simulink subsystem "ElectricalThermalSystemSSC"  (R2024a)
settings: Solver=VariableStepAuto  StartTime=0.0  StopTime=10.0  RelTol=1e-3
undefined symbols (not defined in the file): coolant_pipe_D, coolant_valve_D_ratio_max, coolant_valve_D_ratio_min, coolant_valve_displacement, EnvAirTemp, EnvGrvty, PlantThrEstCmpPwr, PlntThrChArea, PlntThrFanMaxSpd, PlntThrFanMechEff, PlntThrFanVolEff, PlntThrHeaterMaxPwr, PlntThrPipeArea, PlntThrPipeDia, PlntThrPmpMaxSpd, PlntThrRadRamEff, PlntThrRefrigAinit, PlntThrTankArea, PlntThrTankVol, PlntThrValDisp, PlntThrValDratioMax, PlntThrValDratioMin, PlntThrValSplMax, ThrmEM1, ThrmEM2, ThrmEM3, ThrmEM4
libraries: fl_lib x148, nesl_utility x61, SimscapeFluids_lib x25, autolibutils x12
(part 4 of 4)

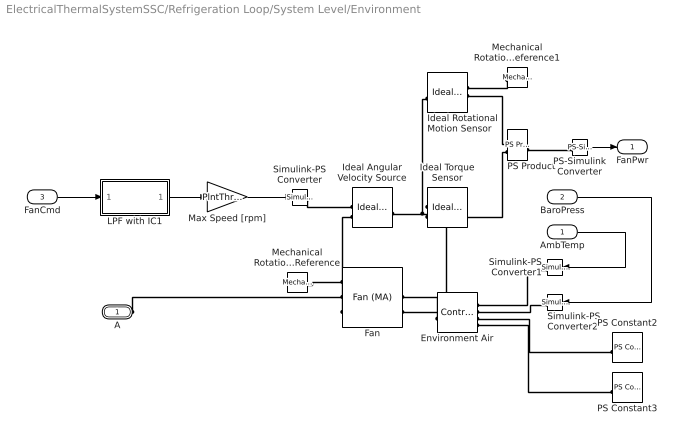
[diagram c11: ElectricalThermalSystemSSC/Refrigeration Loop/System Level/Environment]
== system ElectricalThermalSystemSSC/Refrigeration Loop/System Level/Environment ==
  AmbTemp : Inport
  BaroPress : Inport  Port=2
  FanCmd : Inport  Port=3
  Environment Air : fl_lib/Moist Air/Elements/Controlled Reservoir (MA)  moisture_spec=foundation.enum.moisture_spec.relative_humidity  trace_gas_spec=foundation.enum.trace_gas_spec.mole_fraction  RH_ws=1  area_A=PlntThrRadFanAreaFlw m^2  input_error_spec=foundation.enum.input_range_error.warn
  Fan : SimscapeFluids_lib/Moist Air/Turbomachinery/Fan (MA)  fan_parameterization=fluids.moist_air.turbomachinery.enum.FanParameterization.Nominal  mechanical_power_spec=fluids.moist_air.turbomachinery.enum.FanMechanicalPowerSpec.Efficiency  flow_rate_nominal=0.8 m^3/s  pressure_nominal=PlntThrFanNomP Pa  eta_nominal=PlntThrFanVolEff*PlntThrFanMechEff  power_nominal=1620 W  pressure_max=600 Pa  flow_rate_max=1.5 m^3/s  omega_ref_nominal=1000 rpm  flow_rate_1D_TLU=[.0278, .0556, .0833, .111, .139, .167] m^3/s  pressure_1D_TLU=[6410, 6375, 6018, 5366, 4501, 3609] Pa  eta_1D_TLU=[.257, .394, .453, .47, .459, .415]  power_1D_TLU=[693, 900, 1107, 1267, 1363, 1452] W  omega_ref_1D=3000 rpm  rho_ref_1D=1.2 kg/m^3  omega_threshold_factor=1e-2  omega_dp_TLU=[2400; 3000; 3600] rpm  flow_rate_dp_TLU=[.0278, .0556, .0833, .111, .139, .167] m^3/s  pressure_dp_TLU=[4111, 4010, 3551, 2881, 2167, 1453; 6410, 6375, 6018, 5366, 4501, 3609; 9217, 9285, 9022, 8428, 7552, 6482] Pa  eta_dp_TLU=[.3, .434, .468, .459, .4, .3; .257, .394, .453, .47, .459, .415; .225, .359, .434, .461, .47, .459]  power_dp_TLU=[381, 514, 632, 697, 753, 809; 693, 900, 1107, 1267, 1363, 1452; 1139, 1438, 1732, 2029, 2233, 2358] W  rho_ref_dp=1.2 kg/m^3  omega_q_TLU=[2990; 3450; 3867] rpm  pressure_q_TLU=[31, 62, 93, 124] Pa  flow_rate_q_TLU=[.802, .759, .703, .611; .936, .902, .862, .81; 1.056, 1.027, .994, .956] m^3/s  eta_q_TLU=[.088, .162, .22, .261; .068, .128, .18, .222; .055, .105, .148, .188]  power_q_TLU=[283, 290, 297, 290; 427, 437, 445, 452; 595, 606, 625, 631] W  rho_ref_q=1.2 kg/m^3  diameter_ratio=1  mech_orientation=fluids.moist_air.turbomachinery.enum.FanMechanicalOrientation.Positive  area_A=PlntThrRadFanAreaFlw m^2  area_B=PlntThrRadFanAreaFlw m^2
  Ideal Angular Velocity Source : fl_lib/Mechanical/Mechanical Sources/Ideal Angular Velocity Source
  Ideal Rotational Motion Sensor : fl_lib/Mechanical/Mechanical Sensors/Ideal Rotational Motion Sensor  reference=foundation.enum.MeasurementReference.difference  acceleration_port=false  velocity_port=true  position_port=true  wrap_angle=false  offset=0 rad
  Ideal Torque Sensor : fl_lib/Mechanical/Mechanical Sensors/Ideal Torque Sensor
  LPF with IC1 : Subsystem  mask{wc=0.2, InitCond=0, dataType=off}
      mask prompts: wc "Cutoff frequency, wc [rad/s]"; InitCond "Initial condition, InitCond [same as u]"; dataType "Enforce same input data type"
  Max Speed [rpm] : Gain  Gain=PlntThrFanMaxSpd
  Mechanical Rotational Reference : fl_lib/Mechanical/Rotational Elements/Mechanical Rotational Reference
  Mechanical Rotational Reference1 : fl_lib/Mechanical/Rotational Elements/Mechanical Rotational Reference
  PS Constant2 : fl_lib/Physical Signals/Sources/PS Constant  constant=PlntThrCabRelHInit
  PS Constant3 : fl_lib/Physical Signals/Sources/PS Constant  constant=PlntThrCabCO2Init
  PS Product : fl_lib/Physical Signals/Functions/PS Product
  PS-Simulink Converter : nesl_utility/PS-Simulink Converter  PhysicalDomain=network_engine_domain  SubClassName=ps_output  LeftPortType=input  RightPortType=output  PseudoPeriodic=off  Frequencies=[]  VectorFormat=inherit  Unit=W  AffineConversion=off
  Simulink-PS Converter : nesl_utility/Simulink-PS Converter  PhysicalDomain=network_engine_domain  SubClassName=ps_input  LeftPortType=input  RightPortType=output  PseudoPeriodic=off  Frequencies=[]  NoiseDistribution=none  NoiseParameters=[]  Unit=rpm  AffineConversion=off  FilteringAndDerivatives=provide  SimscapeFilterOrder=1  InputFilterTimeConstant=0.001  UdotUserProvided=0
  Simulink-PS Converter1 : nesl_utility/Simulink-PS Converter  PhysicalDomain=network_engine_domain  SubClassName=ps_input  LeftPortType=input  RightPortType=output  PseudoPeriodic=off  Frequencies=[]  NoiseDistribution=none  NoiseParameters=[]  Unit=K  AffineConversion=on  FilteringAndDerivatives=provide  SimscapeFilterOrder=1  InputFilterTimeConstant=0.001  UdotUserProvided=0
  Simulink-PS Converter2 : nesl_utility/Simulink-PS Converter  PhysicalDomain=network_engine_domain  SubClassName=ps_input  LeftPortType=input  RightPortType=output  PseudoPeriodic=off  Frequencies=[]  NoiseDistribution=none  NoiseParameters=[]  Unit=Pa  AffineConversion=off  FilteringAndDerivatives=provide  SimscapeFilterOrder=1  InputFilterTimeConstant=0.001  UdotUserProvided=0
  A : PMIOPort  Side=Left
  FanPwr : Outport
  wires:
  PS-Simulink Converter/1 -> FanPwr/1
  FanCmd/1 -> LPF with IC1/1(u)
  AmbTemp/1 -> Simulink-PS Converter1/1
  Max Speed [rpm]/1 -> Simulink-PS Converter/1
  BaroPress/1 -> Simulink-PS Converter2/1
  LPF with IC1/1(y) -> Max Speed [rpm]/1
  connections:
  PS-Simulink Converter/LConn1 -- PS Product/RConn1
  PS Product/LConn2 -- Ideal Torque Sensor/RConn2
  PS Product/LConn1 -- Ideal Rotational Motion Sensor/RConn2
  Mechanical Rotational Reference1/LConn1 -- Ideal Rotational Motion Sensor/RConn1
  Ideal Torque Sensor/RConn1 -- Fan/RConn2
  Ideal Rotational Motion Sensor/LConn1 -- Ideal Angular Velocity Source/LConn1 -- Ideal Torque Sensor/LConn1
  PS Constant3/RConn1 -- Environment Air/RConn4
  Environment Air/RConn3 -- PS Constant2/RConn1
  Simulink-PS Converter1/RConn1 -- Environment Air/RConn1
  Environment Air/LConn1 -- Fan/RConn1
  Simulink-PS Converter2/RConn1 -- Environment Air/RConn2
  Ideal Angular Velocity Source/RConn2 -- Mechanical Rotational Reference/LConn1 -- Fan/LConn2
  Simulink-PS Converter/RConn1 -- Ideal Angular Velocity Source/RConn1
  A/RConn1 -- Fan/LConn1

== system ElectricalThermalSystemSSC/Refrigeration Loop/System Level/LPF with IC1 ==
  u : Inport
  Cont LPF IC : autolibutils/Cont LPF IC  wc=wc  aMode=1  dataType=off
  Initial Condition : Constant  Value=InitCond  SampleTime=-1
  y : Outport
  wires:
  Initial Condition/1 -> Cont LPF IC/2
  u/1 -> Cont LPF IC/1
  Cont LPF IC/1 -> y/1

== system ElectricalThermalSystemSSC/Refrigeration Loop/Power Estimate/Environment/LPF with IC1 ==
  u : Inport
  Cont LPF IC : autolibutils/Cont LPF IC  wc=wc  aMode=1  dataType=off
  Initial Condition : Constant  Value=InitCond  SampleTime=-1
  y : Outport
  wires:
  Initial Condition/1 -> Cont LPF IC/2
  u/1 -> Cont LPF IC/1
  Cont LPF IC/1 -> y/1

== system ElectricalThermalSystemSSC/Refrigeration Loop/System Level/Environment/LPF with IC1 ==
  u : Inport
  Cont LPF IC : autolibutils/Cont LPF IC  wc=wc  aMode=1  dataType=off
  Initial Condition : Constant  Value=InitCond  SampleTime=-1
  y : Outport
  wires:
  Initial Condition/1 -> Cont LPF IC/2
  u/1 -> Cont LPF IC/1
  Cont LPF IC/1 -> y/1
